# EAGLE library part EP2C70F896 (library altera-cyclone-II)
EP2C70F896 Auto generated by make-symbol-device-package-bsdl.ulp Rev. 19 Tip: Use split-device-symbol.ulp to generate a Device with multiple small symbols! Read HELP. Source: EP2C70F896.BSD
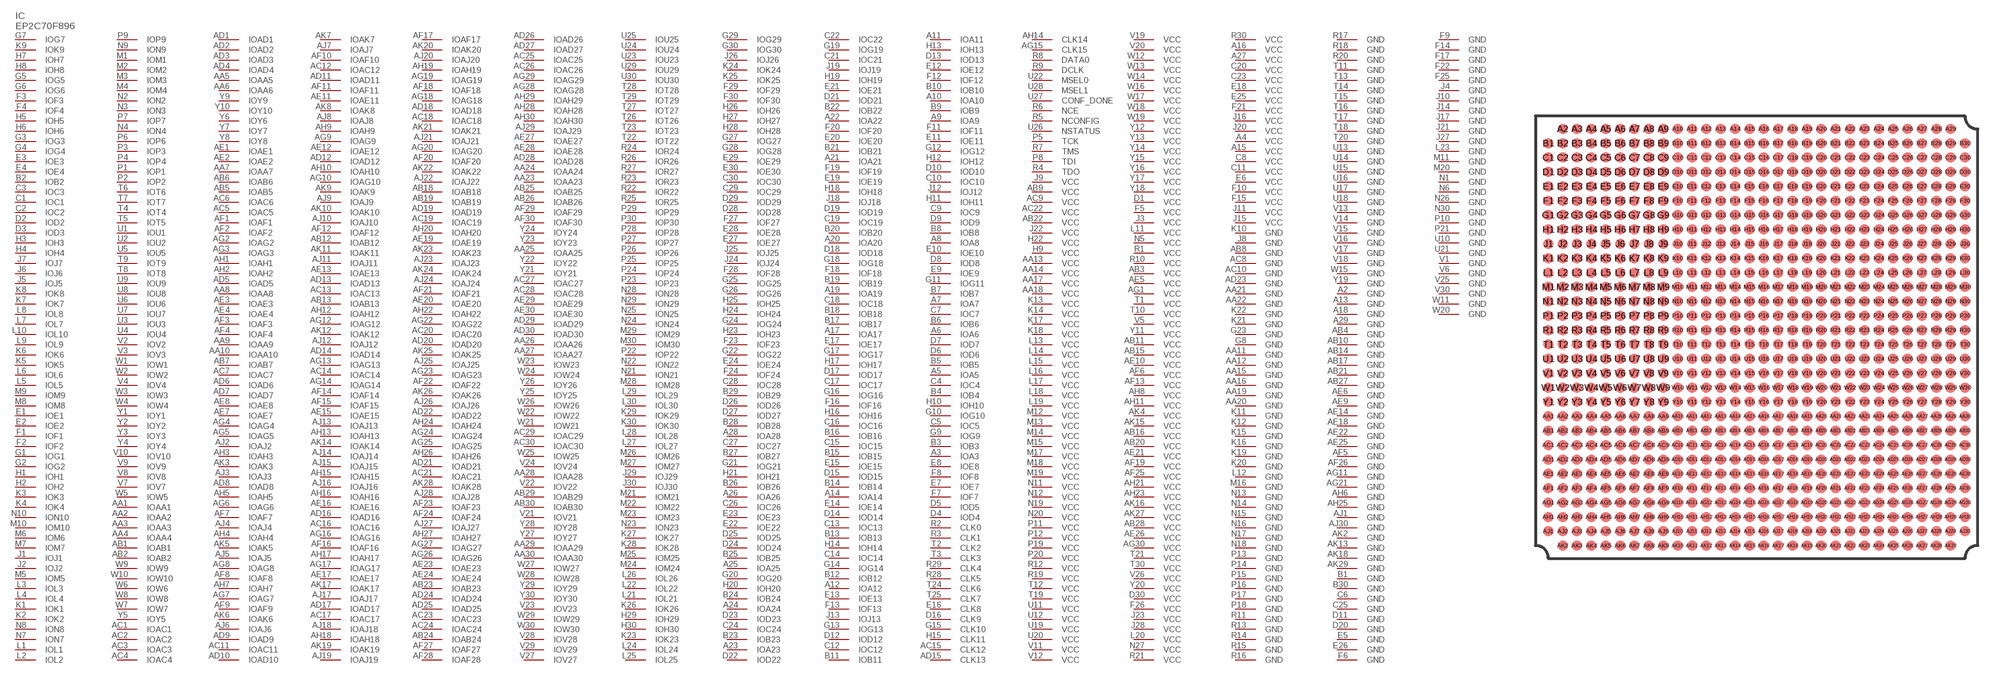
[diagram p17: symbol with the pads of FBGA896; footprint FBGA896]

Designator prefix IC

## EP2C70F896 (MPN: EP2C70F896C8N; OC_FARNELL: 1635092; OC_NEWARK: 51R0573)  [FBGA896]
A2  GND  pwr
A3  IOA3
A4  VCC  pwr
A5  IOA5
A6  IOA6
A7  IOA7
A8  IOA8
A9  IOA9
A10  IOA10
A11  IOA11
A12  IOA12
A13  GND  pwr
A14  IOA14
A15  VCC  pwr
A16  VCC  pwr
A17  IOA17
A18  GND  pwr
A19  IOA19
A20  IOA20
A21  IOA21
A22  IOA22
A23  IOA23
A24  IOA24
A25  IOA25
A26  IOA26
A27  VCC  pwr
A28  IOA28
A29  GND  pwr
AA1  IOAA1
AA2  IOAA2
AA3  IOAA3
AA4  IOAA4
AA5  IOAA5
AA6  IOAA6
AA7  IOAA7
AA8  IOAA8
AA9  IOAA9
AA10  IOAA10
AA11  GND  pwr
AA12  GND  pwr
AA13  VCC  pwr
AA14  VCC  pwr
AA15  GND  pwr
AA16  GND  pwr
AA17  VCC  pwr
AA18  VCC  pwr
AA19  GND  pwr
AA20  GND  pwr
AA21  GND  pwr
AA22  GND  pwr
AA23  IOAA23
AA24  IOAA24
AA25  IOAA25
AA26  IOAA26
AA27  IOAA27
AA28  IOAA28
AA29  IOAA29
AA30  IOAA30
AB1  IOAB1
AB2  IOAB2
AB3  VCC  pwr
AB4  GND  pwr
AB5  IOAB5
AB6  IOAB6
AB7  IOAB7
AB8  GND  pwr
AB9  VCC  pwr
AB10  GND  pwr
AB11  VCC  pwr
AB12  IOAB12
AB13  IOAB13
AB14  GND  pwr
AB15  VCC  pwr
AB16  VCC  pwr
AB17  GND  pwr
AB18  IOAB18
AB19  IOAB19
AB20  VCC  pwr
AB21  GND  pwr
AB22  VCC  pwr
AB23  IOAB23
AB24  IOAB24
AB25  IOAB25
AB26  IOAB26
AB27  GND  pwr
AB28  VCC  pwr
AB29  IOAB29
AB30  IOAB30
AC1  IOAC1
AC2  IOAC2
AC3  IOAC3
AC4  IOAC4
AC5  IOAC5
AC6  IOAC6
AC7  IOAC7
AC8  GND  pwr
AC9  VCC  pwr
AC10  GND  pwr
AC11  IOAC11
AC12  IOAC12
AC13  IOAC13
AC14  IOAC14
AC15  CLK12
AC16  IOAC16
AC17  IOAC17
AC18  IOAC18
AC19  IOAC19
AC20  IOAC20
AC21  IOAC21
AC22  VCC  pwr
AC23  IOAC23
AC24  IOAC24
AC25  IOAC25
AC26  IOAC26
AC27  IOAC27
AC28  IOAC28
AC29  IOAC29
AC30  IOAC30
AD1  IOAD1
AD2  IOAD2
AD3  IOAD3
AD4  IOAD4
AD5  IOAD5
AD6  IOAD6
AD7  IOAD7
AD8  IOAD8
AD9  IOAD9
AD10  IOAD10
AD11  IOAD11
AD12  IOAD12
AD13  IOAD13
AD14  IOAD14
AD15  CLK13
AD16  IOAD16
AD17  IOAD17
AD18  IOAD18
AD19  IOAD19
AD20  IOAD20
AD21  IOAD21
AD22  IOAD22
AD23  GND  pwr
AD24  IOAD24
AD25  IOAD25
AD26  IOAD26
AD27  IOAD27
AD28  IOAD28
AD29  IOAD29
AD30  IOAD30
AE1  IOAE1
AE2  IOAE2
AE3  IOAE3
AE4  IOAE4
AE5  VCC  pwr
AE6  GND  pwr
AE7  IOAE7
AE8  IOAE8
AE9  GND  pwr
AE10  VCC  pwr
AE11  IOAE11
AE12  IOAE12
AE13  IOAE13
AE14  GND  pwr
AE15  IOAE15
AE16  IOAE16
AE17  IOAE17
AE18  GND  pwr
AE19  IOAE19
AE20  IOAE20
AE21  VCC  pwr
AE22  GND  pwr
AE23  IOAE23
AE24  IOAE24
AE25  GND  pwr
AE26  VCC  pwr
AE27  IOAE27
AE28  IOAE28
AE29  IOAE29
AE30  IOAE30
AF1  IOAF1
AF2  IOAF2
AF3  IOAF3
AF4  IOAF4
AF5  GND  pwr
AF6  VCC  pwr
AF7  IOAF7
AF8  IOAF8
AF9  IOAF9
AF10  IOAF10
AF11  IOAF11
AF12  IOAF12
AF13  VCC  pwr
AF14  IOAF14
AF15  IOAF15
AF16  IOAF16
AF17  IOAF17
AF18  IOAF18
AF19  VCC  pwr
AF20  IOAF20
AF21  IOAF21
AF22  IOAF22
AF23  IOAF23
AF24  IOAF24
AF25  VCC  pwr
AF26  GND  pwr
AF27  IOAF27
AF28  IOAF28
AF29  IOAF29
AF30  IOAF30
AG1  VCC  pwr
AG2  IOAG2
AG3  IOAG3
AG4  IOAG4
AG5  IOAG5
AG6  IOAG6
AG7  IOAG7
AG8  IOAG8
AG9  IOAG9
AG10  IOAG10
AG11  GND  pwr
AG12  IOAG12
AG13  IOAG13
AG14  IOAG14
AG15  CLK15
AG16  IOAG16
AG17  IOAG17
AG18  IOAG18
AG19  IOAG19
AG20  IOAG20
AG21  GND  pwr
AG22  IOAG22
AG23  IOAG23
AG24  IOAG24
AG25  IOAG25
AG26  IOAG26
AG27  IOAG27
AG28  IOAG28
AG29  IOAG29
AG30  VCC  pwr
AH1  IOAH1
AH2  IOAH2
AH3  IOAH3
AH4  IOAH4
AH5  IOAH5
AH6  GND  pwr
AH7  IOAH7
AH8  VCC  pwr
AH9  IOAH9
AH10  IOAH10
AH11  VCC  pwr
AH12  IOAH12
AH13  IOAH13
AH14  CLK14
AH15  IOAH15
AH16  IOAH16
AH17  IOAH17
AH18  IOAH18
AH19  IOAH19
AH20  IOAH20
AH21  VCC  pwr
AH22  IOAH22
AH23  VCC  pwr
AH24  IOAH24
AH25  GND  pwr
AH26  IOAH26
AH27  IOAH27
AH28  IOAH28
AH29  IOAH29
AH30  IOAH30
AJ1  GND  pwr
AJ2  IOAJ2
AJ3  IOAJ3
AJ4  IOAJ4
AJ5  IOAJ5
AJ6  IOAJ6
AJ7  IOAJ7
AJ8  IOAJ8
AJ9  IOAJ9
AJ10  IOAJ10
AJ11  IOAJ11
AJ12  IOAJ12
AJ13  IOAJ13
AJ14  IOAJ14
AJ15  IOAJ15
AJ16  IOAJ16
AJ17  IOAJ17
AJ18  IOAJ18
AJ19  IOAJ19
AJ20  IOAJ20
AJ21  IOAJ21
AJ22  IOAJ22
AJ23  IOAJ23
AJ24  IOAJ24
AJ25  IOAJ25
AJ26  IOAJ26
AJ27  IOAJ27
AJ28  IOAJ28
AJ29  IOAJ29
AJ30  GND  pwr
AK2  GND  pwr
AK3  IOAK3
AK4  VCC  pwr
AK5  IOAK5
AK6  IOAK6
AK7  IOAK7
AK8  IOAK8
AK9  IOAK9
AK10  IOAK10
AK11  IOAK11
AK12  IOAK12
AK13  GND  pwr
AK14  IOAK14
AK15  VCC  pwr
AK16  VCC  pwr
AK17  IOAK17
AK18  GND  pwr
AK19  IOAK19
AK20  IOAK20
AK21  IOAK21
AK22  IOAK22
AK23  IOAK23
AK24  IOAK24
AK25  IOAK25
AK26  IOAK26
AK27  VCC  pwr
AK28  IOAK28
AK29  GND  pwr
B1  GND  pwr
B2  IOB2
B3  IOB3
B4  IOB4
B5  IOB5
B6  IOB6
B7  IOB7
B8  IOB8
B9  IOB9
B10  IOB10
B11  IOB11
B12  IOB12
B13  IOB13
B14  IOB14
B15  IOB15
B16  IOB16
B17  IOB17
B18  IOB18
B19  IOB19
B20  IOB20
B21  IOB21
B22  IOB22
B23  IOB23
B24  IOB24
B25  IOB25
B26  IOB26
B27  IOB27
B28  IOB28
B29  IOB29
B30  GND  pwr
C1  IOC1
C2  IOC2
C3  IOC3
C4  IOC4
C5  IOC5
C6  GND  pwr
C7  IOC7
C8  VCC  pwr
C9  IOC9
C10  IOC10
C11  VCC  pwr
C12  IOC12
C13  IOC13
C14  IOC14
C15  IOC15
C16  IOC16
C17  IOC17
C18  IOC18
C19  IOC19
C20  VCC  pwr
C21  IOC21
C22  IOC22
C23  VCC  pwr
C24  IOC24
C25  GND  pwr
C26  IOC26
C27  IOC27
C28  IOC28
C29  IOC29
C30  IOC30
D1  VCC  pwr
D2  IOD2
D3  IOD3
D4  IOD4
D5  IOD5
D6  IOD6
D7  IOD7
D8  IOD8
D9  IOD9
D10  IOD10
D11  GND  pwr
D12  IOD12
D13  IOD13
D14  IOD14
D15  IOD15
D16  CLK9
D17  IOD17
D18  IOD18
D19  IOD19
D20  GND  pwr
D21  IOD21
D22  IOD22
D23  IOD23
D24  IOD24
D25  IOD25
D26  IOD26
D27  IOD27
D28  IOD28
D29  IOD29
D30  VCC  pwr
E1  IOE1
E2  IOE2
E3  IOE3
E4  IOE4
E5  GND  pwr
E6  VCC  pwr
E7  IOE7
E8  IOE8
E9  IOE9
E10  IOE10
E11  IOE11
E12  IOE12
E13  IOE13
E14  IOE14
E15  IOE15
E16  CLK8
E17  IOE17
E18  VCC  pwr
E19  IOE19
E20  IOE20
E21  IOE21
E22  IOE22
E23  IOE23
E24  IOE24
E25  VCC  pwr
E26  GND  pwr
E27  IOE27
E28  IOE28
E29  IOE29
E30  IOE30
F1  IOF1
F2  IOF2
F3  IOF3
F4  IOF4
F5  VCC  pwr
F6  GND  pwr
F7  IOF7
F8  IOF8
F9  GND  pwr
F10  VCC  pwr
F11  IOF11
F12  IOF12
F13  IOF13
F14  GND  pwr
F15  VCC  pwr
F16  IOF16
F17  GND  pwr
F18  IOF18
F19  IOF19
F20  IOF20
F21  VCC  pwr
F22  GND  pwr
F23  IOF23
F24  IOF24
F25  GND  pwr
F26  VCC  pwr
F27  IOF27
F28  IOF28
F29  IOF29
F30  IOF30
G1  IOG1
G2  IOG2
G3  IOG3
G4  IOG4
G5  IOG5
G6  IOG6
G7  IOG7  out
G8  GND  pwr
G9  IOG9
G10  IOG10
G11  IOG11
G12  IOG12
G13  IOG13
G14  IOG14
G15  CLK10
G16  IOG16
G17  IOG17
G18  IOG18
G19  IOG19
G20  IOG20
G21  IOG21
G22  IOG22
G23  GND  pwr
G24  IOG24
G25  IOG25
G26  IOG26
G27  IOG27
G28  IOG28
G29  IOG29
G30  IOG30
H1  IOH1
H2  IOH2
H3  IOH3
H4  IOH4
H5  IOH5
H6  IOH6
H7  IOH7
H8  IOH8
H9  VCC  pwr
H10  IOH10
H11  IOH11
H12  IOH12
H13  IOH13
H14  IOH14
H15  CLK11
H16  IOH16
H17  IOH17
H18  IOH18
H19  IOH19
H20  IOH20
H21  IOH21
H22  VCC  pwr
H23  IOH23
H24  IOH24
H25  IOH25
H26  IOH26
H27  IOH27
H28  IOH28
H29  IOH29
H30  IOH30
J1  IOJ1
J2  IOJ2
J3  VCC  pwr
J4  GND  pwr
J5  IOJ5
J6  IOJ6
J7  IOJ7
J8  GND  pwr
J9  VCC  pwr
J10  GND  pwr
J11  VCC  pwr
J12  IOJ12
J13  IOJ13
J14  GND  pwr
J15  VCC  pwr
J16  VCC  pwr
J17  GND  pwr
J18  IOJ18
J19  IOJ19
J20  VCC  pwr
J21  GND  pwr
J22  VCC  pwr
J23  VCC  pwr
J24  IOJ24
J25  IOJ25
J26  IOJ26
J27  GND  pwr
J28  VCC  pwr
J29  IOJ29
J30  IOJ30
K1  IOK1
K2  IOK2
K3  IOK3
K4  IOK4
K5  IOK5
K6  IOK6
K7  IOK7
K8  IOK8
K9  IOK9  out
K10  GND  pwr
K11  GND  pwr
K12  GND  pwr
K13  VCC  pwr
K14  VCC  pwr
K15  GND  pwr
K16  GND  pwr
K17  VCC  pwr
K18  VCC  pwr
K19  GND  pwr
K20  GND  pwr
K21  GND  pwr
K22  GND  pwr
K23  IOK23
K24  IOK24
K25  IOK25
K26  IOK26
K27  IOK27
K28  IOK28
K29  IOK29
K30  IOK30
L1  IOL1
L2  IOL2
L3  IOL3
L4  IOL4
L5  IOL5
L6  IOL6
L7  IOL7
L8  IOL8
L9  IOL9
L10  IOL10
L11  VCC  pwr
L12  GND  pwr
L13  VCC  pwr
L14  VCC  pwr
L15  VCC  pwr
L16  VCC  pwr
L17  VCC  pwr
L18  VCC  pwr
L19  VCC  pwr
L20  VCC  pwr
L21  IOL21
L22  IOL22
L23  GND  pwr
L24  IOL24
L25  IOL25
L26  IOL26
L27  IOL27
L28  IOL28
L29  IOL29
L30  IOL30
M1  IOM1
M2  IOM2
M3  IOM3
M4  IOM4
M5  IOM5
M6  IOM6
M7  IOM7
M8  IOM8
M9  IOM9
M10  IOM10
M11  GND  pwr
M12  VCC  pwr
M13  VCC  pwr
M14  VCC  pwr
M15  VCC  pwr
M16  GND  pwr
M17  VCC  pwr
M18  VCC  pwr
M19  VCC  pwr
M20  GND  pwr
M21  IOM21
M22  IOM22
M23  IOM23
M24  IOM24
M25  IOM25
M26  IOM26
M27  IOM27
M28  IOM28
M29  IOM29
M30  IOM30
N1  GND  pwr
N2  ION2
N3  ION3
N4  ION4
N5  VCC  pwr
N6  GND  pwr
N7  ION7
N8  ION8
N9  ION9
N10  ION10
N11  VCC  pwr
N12  VCC  pwr
N13  GND  pwr
N14  GND  pwr
N15  GND  pwr
N16  GND  pwr
N17  GND  pwr
N18  GND  pwr
N19  VCC  pwr
N20  VCC  pwr
N21  ION21
N22  ION22
N23  ION23
N24  ION24
N25  ION25
N26  GND  pwr
N27  VCC  pwr
N28  ION28
N29  ION29
N30  GND  pwr
P1  IOP1
P2  IOP2
P3  IOP3
P4  IOP4
P5  TCK  in
P6  IOP6
P7  IOP7
P8  TDI  in
P9  IOP9
P10  GND  pwr
P11  VCC  pwr
P12  VCC  pwr
P13  GND  pwr
P14  GND  pwr
P15  GND  pwr
P16  GND  pwr
P17  GND  pwr
P18  GND  pwr
P19  VCC  pwr
P20  VCC  pwr
P21  GND  pwr
P22  IOP22
P23  IOP23
P24  IOP24
P25  IOP25
P26  IOP26
P27  IOP27
P28  IOP28
P29  IOP29
P30  IOP30
R1  VCC  pwr
R2  CLK0
R3  CLK1
R4  TDO  out
R5  NCONFIG  in
R6  NCE  in
R7  TMS  in
R8  DATA0
R9  DCLK
R10  VCC  pwr
R11  GND  pwr
R12  VCC  pwr
R13  GND  pwr
R14  GND  pwr
R15  GND  pwr
R16  GND  pwr
R17  GND  pwr
R18  GND  pwr
R19  VCC  pwr
R20  GND  pwr
R21  VCC  pwr
R22  IOR22
R23  IOR23
R24  IOR24
R25  IOR25
R26  IOR26
R27  IOR27
R28  CLK5
R29  CLK4
R30  VCC  pwr
T1  VCC  pwr
T2  CLK2
T3  CLK3
T4  IOT4
T5  IOT5
T6  IOT6
T7  IOT7
T8  IOT8
T9  IOT9
T10  VCC  pwr
T11  GND  pwr
T12  VCC  pwr
T13  GND  pwr
T14  GND  pwr
T15  GND  pwr
T16  GND  pwr
T17  GND  pwr
T18  GND  pwr
T19  VCC  pwr
T20  GND  pwr
T21  VCC  pwr
T22  IOT22
T23  IOT23
T24  CLK6
T25  CLK7
T26  IOT26
T27  IOT27
T28  IOT28
T29  IOT29
T30  VCC  pwr
U1  IOU1
U2  IOU2
U3  IOU3
U4  IOU4
U5  IOU5
U6  IOU6
U7  IOU7
U8  IOU8
U9  IOU9
U10  GND  pwr
U11  VCC  pwr
U12  VCC  pwr
U13  GND  pwr
U14  GND  pwr
U15  GND  pwr
U16  GND  pwr
U17  GND  pwr
U18  GND  pwr
U19  VCC  pwr
U20  VCC  pwr
U21  GND  pwr
U22  MSEL0  in
U23  IOU23
U24  IOU24
U25  IOU25
U26  NSTATUS  in
U27  CONF_DONE  in
U28  MSEL1  in
U29  IOU29
U30  IOU30
V1  GND  pwr
V2  IOV2
V3  IOV3
V4  IOV4
V5  VCC  pwr
V6  GND  pwr
V7  IOV7
V8  IOV8
V9  IOV9
V10  IOV10
V11  VCC  pwr
V12  VCC  pwr
V13  GND  pwr
V14  GND  pwr
V15  GND  pwr
V16  GND  pwr
V17  GND  pwr
V18  GND  pwr
V19  VCC  pwr
V20  VCC  pwr
V21  IOV21
V22  IOV22
V23  IOV23
V24  IOV24
V25  GND  pwr
V26  VCC  pwr
V27  IOV27
V28  IOV28
V29  IOV29
V30  GND  pwr
W1  IOW1
W2  IOW2
W3  IOW3
W4  IOW4
W5  IOW5
W6  IOW6
W7  IOW7
W8  IOW8
W9  IOW9
W10  IOW10
W11  GND  pwr
W12  VCC  pwr
W13  VCC  pwr
W14  VCC  pwr
W15  GND  pwr
W16  VCC  pwr
W17  VCC  pwr
W18  VCC  pwr
W19  VCC  pwr
W20  GND  pwr
W21  IOW21
W22  IOW22
W23  IOW23
W24  IOW24
W25  IOW25
W26  IOW26
W27  IOW27
W28  IOW28
W29  IOW29
W30  IOW30
Y1  IOY1
Y2  IOY2
Y3  IOY3
Y4  IOY4
Y5  IOY5
Y6  IOY6
Y7  IOY7
Y8  IOY8
Y9  IOY9
Y10  IOY10
Y11  VCC  pwr
Y12  VCC  pwr
Y13  VCC  pwr
Y14  VCC  pwr
Y15  VCC  pwr
Y16  VCC  pwr
Y17  VCC  pwr
Y18  VCC  pwr
Y19  GND  pwr
Y20  VCC  pwr
Y21  IOY21
Y22  IOY22
Y23  IOY23
Y24  IOY24
Y25  IOY25
Y26  IOY26
Y27  IOY27
Y28  IOY28
Y29  IOY29
Y30  IOY30

## Footprint FBGA896 (pad centres in mm)
EP2C70F896 Auto generated by make-symbol-device-package-bsdl.ulp Rev. 19 Source: EP2C70F896.BSD www.altera.com .. cyc2_cii51015.pdf
smd 0.7 x 0.7: A2 -13.5,14.5; A3 -12.5,14.5; A4 -11.5,14.5; A5 -10.5,14.5; A6 -9.5,14.5; A7 -8.5,14.5; A8 -7.5,14.5; A9 -6.5,14.5; A10 -5.5,14.5; A11 -4.5,14.5; A12 -3.5,14.5; A13 -2.5,14.5; A14 -1.5,14.5; A15 -0.5,14.5; A16 0.5,14.5; A17 1.5,14.5; A18 2.5,14.5; A19 3.5,14.5; A20 4.5,14.5; A21 5.5,14.5; A22 6.5,14.5; A23 7.5,14.5; A24 8.5,14.5; A25 9.5,14.5; A26 10.5,14.5; A27 11.5,14.5; A28 12.5,14.5; A29 13.5,14.5; AA1 -14.5,-5.5; AA2 -13.5,-5.5; AA3 -12.5,-5.5; AA4 -11.5,-5.5; AA5 -10.5,-5.5; AA6 -9.5,-5.5; AA7 -8.5,-5.5; AA8 -7.5,-5.5; AA9 -6.5,-5.5; AA10 -5.5,-5.5; AA11 -4.5,-5.5; AA12 -3.5,-5.5; AA13 -2.5,-5.5; AA14 -1.5,-5.5; AA15 -0.5,-5.5; AA16 0.5,-5.5; AA17 1.5,-5.5; AA18 2.5,-5.5; AA19 3.5,-5.5; AA20 4.5,-5.5; AA21 5.5,-5.5; AA22 6.5,-5.5; AA23 7.5,-5.5; AA24 8.5,-5.5; AA25 9.5,-5.5; AA26 10.5,-5.5; AA27 11.5,-5.5; AA28 12.5,-5.5; AA29 13.5,-5.5; AA30 14.5,-5.5; AB1 -14.5,-6.5; AB2 -13.5,-6.5; AB3 -12.5,-6.5; AB4 -11.5,-6.5; AB5 -10.5,-6.5; AB6 -9.5,-6.5; AB7 -8.5,-6.5; AB8 -7.5,-6.5; AB9 -6.5,-6.5; AB10 -5.5,-6.5; AB11 -4.5,-6.5; AB12 -3.5,-6.5; AB13 -2.5,-6.5; AB14 -1.5,-6.5; AB15 -0.5,-6.5; AB16 0.5,-6.5; AB17 1.5,-6.5; AB18 2.5,-6.5; AB19 3.5,-6.5; AB20 4.5,-6.5; AB21 5.5,-6.5; AB22 6.5,-6.5; AB23 7.5,-6.5; AB24 8.5,-6.5; AB25 9.5,-6.5; AB26 10.5,-6.5; AB27 11.5,-6.5; AB28 12.5,-6.5; AB29 13.5,-6.5; AB30 14.5,-6.5; AC1 -14.5,-7.5; AC2 -13.5,-7.5; AC3 -12.5,-7.5; AC4 -11.5,-7.5; AC5 -10.5,-7.5; AC6 -9.5,-7.5; AC7 -8.5,-7.5; AC8 -7.5,-7.5; AC9 -6.5,-7.5; AC10 -5.5,-7.5; AC11 -4.5,-7.5; AC12 -3.5,-7.5; AC13 -2.5,-7.5; AC14 -1.5,-7.5; AC15 -0.5,-7.5; AC16 0.5,-7.5; AC17 1.5,-7.5; AC18 2.5,-7.5; AC19 3.5,-7.5; AC20 4.5,-7.5; AC21 5.5,-7.5; AC22 6.5,-7.5; AC23 7.5,-7.5; AC24 8.5,-7.5; AC25 9.5,-7.5; AC26 10.5,-7.5; AC27 11.5,-7.5; AC28 12.5,-7.5; AC29 13.5,-7.5; AC30 14.5,-7.5; AD1 -14.5,-8.5; AD2 -13.5,-8.5; AD3 -12.5,-8.5; AD4 -11.5,-8.5; AD5 -10.5,-8.5; AD6 -9.5,-8.5; AD7 -8.5,-8.5; AD8 -7.5,-8.5; AD9 -6.5,-8.5; AD10 -5.5,-8.5; AD11 -4.5,-8.5; AD12 -3.5,-8.5; AD13 -2.5,-8.5; AD14 -1.5,-8.5; AD15 -0.5,-8.5; AD16 0.5,-8.5; AD17 1.5,-8.5; AD18 2.5,-8.5; AD19 3.5,-8.5; AD20 4.5,-8.5; AD21 5.5,-8.5; AD22 6.5,-8.5; AD23 7.5,-8.5; AD24 8.5,-8.5; AD25 9.5,-8.5; AD26 10.5,-8.5; AD27 11.5,-8.5; AD28 12.5,-8.5; AD29 13.5,-8.5; AD30 14.5,-8.5; AE1 -14.5,-9.5; AE2 -13.5,-9.5; AE3 -12.5,-9.5; AE4 -11.5,-9.5; AE5 -10.5,-9.5; AE6 -9.5,-9.5; AE7 -8.5,-9.5; AE8 -7.5,-9.5; AE9 -6.5,-9.5; AE10 -5.5,-9.5; AE11 -4.5,-9.5; AE12 -3.5,-9.5; AE13 -2.5,-9.5; AE14 -1.5,-9.5; AE15 -0.5,-9.5; AE16 0.5,-9.5; AE17 1.5,-9.5; AE18 2.5,-9.5; AE19 3.5,-9.5; AE20 4.5,-9.5; AE21 5.5,-9.5; AE22 6.5,-9.5; AE23 7.5,-9.5; AE24 8.5,-9.5; AE25 9.5,-9.5; AE26 10.5,-9.5; AE27 11.5,-9.5; AE28 12.5,-9.5; AE29 13.5,-9.5; AE30 14.5,-9.5; AF1 -14.5,-10.5; AF2 -13.5,-10.5; AF3 -12.5,-10.5; AF4 -11.5,-10.5; AF5 -10.5,-10.5; AF6 -9.5,-10.5; AF7 -8.5,-10.5; AF8 -7.5,-10.5; AF9 -6.5,-10.5; AF10 -5.5,-10.5; AF11 -4.5,-10.5; AF12 -3.5,-10.5; AF13 -2.5,-10.5; AF14 -1.5,-10.5; AF15 -0.5,-10.5; AF16 0.5,-10.5; AF17 1.5,-10.5; AF18 2.5,-10.5; AF19 3.5,-10.5; AF20 4.5,-10.5; AF21 5.5,-10.5; AF22 6.5,-10.5; AF23 7.5,-10.5; AF24 8.5,-10.5; AF25 9.5,-10.5; AF26 10.5,-10.5; AF27 11.5,-10.5; AF28 12.5,-10.5; AF29 13.5,-10.5; AF30 14.5,-10.5; AG1 -14.5,-11.5; AG2 -13.5,-11.5; AG3 -12.5,-11.5; AG4 -11.5,-11.5; AG5 -10.5,-11.5; AG6 -9.5,-11.5; AG7 -8.5,-11.5; AG8 -7.5,-11.5; AG9 -6.5,-11.5; AG10 -5.5,-11.5; AG11 -4.5,-11.5; AG12 -3.5,-11.5; AG13 -2.5,-11.5; AG14 -1.5,-11.5; AG15 -0.5,-11.5; AG16 0.5,-11.5; AG17 1.5,-11.5; AG18 2.5,-11.5; AG19 3.5,-11.5; AG20 4.5,-11.5; AG21 5.5,-11.5; AG22 6.5,-11.5; AG23 7.5,-11.5; AG24 8.5,-11.5; AG25 9.5,-11.5; AG26 10.5,-11.5; AG27 11.5,-11.5; AG28 12.5,-11.5; AG29 13.5,-11.5; AG30 14.5,-11.5; AH1 -14.5,-12.5; AH2 -13.5,-12.5; AH3 -12.5,-12.5; AH4 -11.5,-12.5; AH5 -10.5,-12.5; AH6 -9.5,-12.5; AH7 -8.5,-12.5; AH8 -7.5,-12.5; AH9 -6.5,-12.5; AH10 -5.5,-12.5; AH11 -4.5,-12.5; AH12 -3.5,-12.5; AH13 -2.5,-12.5; AH14 -1.5,-12.5; AH15 -0.5,-12.5; AH16 0.5,-12.5; AH17 1.5,-12.5; AH18 2.5,-12.5; AH19 3.5,-12.5; AH20 4.5,-12.5; AH21 5.5,-12.5; AH22 6.5,-12.5; AH23 7.5,-12.5; AH24 8.5,-12.5; AH25 9.5,-12.5; AH26 10.5,-12.5; AH27 11.5,-12.5; AH28 12.5,-12.5; AH29 13.5,-12.5; AH30 14.5,-12.5; AJ1 -14.5,-13.5; AJ2 -13.5,-13.5; AJ3 -12.5,-13.5; AJ4 -11.5,-13.5; AJ5 -10.5,-13.5; AJ6 -9.5,-13.5; AJ7 -8.5,-13.5; AJ8 -7.5,-13.5; AJ9 -6.5,-13.5; AJ10 -5.5,-13.5; AJ11 -4.5,-13.5; AJ12 -3.5,-13.5; AJ13 -2.5,-13.5; AJ14 -1.5,-13.5; AJ15 -0.5,-13.5; AJ16 0.5,-13.5; AJ17 1.5,-13.5; AJ18 2.5,-13.5; AJ19 3.5,-13.5; AJ20 4.5,-13.5; AJ21 5.5,-13.5; AJ22 6.5,-13.5; AJ23 7.5,-13.5; AJ24 8.5,-13.5; AJ25 9.5,-13.5; AJ26 10.5,-13.5; AJ27 11.5,-13.5; AJ28 12.5,-13.5; AJ29 13.5,-13.5; AJ30 14.5,-13.5; AK2 -13.5,-14.5; AK3 -12.5,-14.5; AK4 -11.5,-14.5; AK5 -10.5,-14.5; AK6 -9.5,-14.5; AK7 -8.5,-14.5; AK8 -7.5,-14.5; AK9 -6.5,-14.5; AK10 -5.5,-14.5; AK11 -4.5,-14.5; AK12 -3.5,-14.5; AK13 -2.5,-14.5; AK14 -1.5,-14.5; AK15 -0.5,-14.5; AK16 0.5,-14.5; AK17 1.5,-14.5; AK18 2.5,-14.5; AK19 3.5,-14.5; AK20 4.5,-14.5; AK21 5.5,-14.5; AK22 6.5,-14.5; AK23 7.5,-14.5; AK24 8.5,-14.5; AK25 9.5,-14.5; AK26 10.5,-14.5; AK27 11.5,-14.5; AK28 12.5,-14.5; AK29 13.5,-14.5; B1 -14.5,13.5; B2 -13.5,13.5; B3 -12.5,13.5; B4 -11.5,13.5; B5 -10.5,13.5; B6 -9.5,13.5; B7 -8.5,13.5; B8 -7.5,13.5; B9 -6.5,13.5; B10 -5.5,13.5; B11 -4.5,13.5; B12 -3.5,13.5; B13 -2.5,13.5; B14 -1.5,13.5; B15 -0.5,13.5; B16 0.5,13.5; B17 1.5,13.5; B18 2.5,13.5; B19 3.5,13.5; B20 4.5,13.5; B21 5.5,13.5; B22 6.5,13.5; B23 7.5,13.5; B24 8.5,13.5; B25 9.5,13.5; B26 10.5,13.5; B27 11.5,13.5; B28 12.5,13.5; B29 13.5,13.5; B30 14.5,13.5; C1 -14.5,12.5; C2 -13.5,12.5; C3 -12.5,12.5; C4 -11.5,12.5; C5 -10.5,12.5; C6 -9.5,12.5; C7 -8.5,12.5; C8 -7.5,12.5; C9 -6.5,12.5; C10 -5.5,12.5; C11 -4.5,12.5; C12 -3.5,12.5; C13 -2.5,12.5; C14 -1.5,12.5; C15 -0.5,12.5; C16 0.5,12.5; C17 1.5,12.5; C18 2.5,12.5; C19 3.5,12.5; C20 4.5,12.5; C21 5.5,12.5; C22 6.5,12.5; C23 7.5,12.5; C24 8.5,12.5; C25 9.5,12.5; C26 10.5,12.5; C27 11.5,12.5; C28 12.5,12.5; C29 13.5,12.5; C30 14.5,12.5; D1 -14.5,11.5; D2 -13.5,11.5; D3 -12.5,11.5; D4 -11.5,11.5; D5 -10.5,11.5; D6 -9.5,11.5; D7 -8.5,11.5; D8 -7.5,11.5; D9 -6.5,11.5; D10 -5.5,11.5; D11 -4.5,11.5; D12 -3.5,11.5; D13 -2.5,11.5; D14 -1.5,11.5; D15 -0.5,11.5; D16 0.5,11.5; D17 1.5,11.5; D18 2.5,11.5; D19 3.5,11.5; D20 4.5,11.5; D21 5.5,11.5; D22 6.5,11.5; D23 7.5,11.5; D24 8.5,11.5; D25 9.5,11.5; D26 10.5,11.5; D27 11.5,11.5; D28 12.5,11.5; D29 13.5,11.5; D30 14.5,11.5; E1 -14.5,10.5; E2 -13.5,10.5; E3 -12.5,10.5; E4 -11.5,10.5; E5 -10.5,10.5; E6 -9.5,10.5; E7 -8.5,10.5; E8 -7.5,10.5; E9 -6.5,10.5; E10 -5.5,10.5; E11 -4.5,10.5; E12 -3.5,10.5; E13 -2.5,10.5; E14 -1.5,10.5; E15 -0.5,10.5; E16 0.5,10.5; E17 1.5,10.5; E18 2.5,10.5; E19 3.5,10.5; E20 4.5,10.5; E21 5.5,10.5; E22 6.5,10.5; E23 7.5,10.5; E24 8.5,10.5; E25 9.5,10.5; E26 10.5,10.5; E27 11.5,10.5; E28 12.5,10.5; E29 13.5,10.5; E30 14.5,10.5; F1 -14.5,9.5; F2 -13.5,9.5; F3 -12.5,9.5; F4 -11.5,9.5; F5 -10.5,9.5; F6 -9.5,9.5; F7 -8.5,9.5; F8 -7.5,9.5; F9 -6.5,9.5; F10 -5.5,9.5; F11 -4.5,9.5; F12 -3.5,9.5; F13 -2.5,9.5; F14 -1.5,9.5; F15 -0.5,9.5; F16 0.5,9.5; F17 1.5,9.5; F18 2.5,9.5; F19 3.5,9.5; F20 4.5,9.5; F21 5.5,9.5; F22 6.5,9.5; F23 7.5,9.5; F24 8.5,9.5; F25 9.5,9.5; F26 10.5,9.5; F27 11.5,9.5; F28 12.5,9.5; F29 13.5,9.5; F30 14.5,9.5; G1 -14.5,8.5; G2 -13.5,8.5; G3 -12.5,8.5; G4 -11.5,8.5; G5 -10.5,8.5; G6 -9.5,8.5; G7 -8.5,8.5; G8 -7.5,8.5; G9 -6.5,8.5; G10 -5.5,8.5; G11 -4.5,8.5; G12 -3.5,8.5; G13 -2.5,8.5; G14 -1.5,8.5; G15 -0.5,8.5; G16 0.5,8.5; G17 1.5,8.5; G18 2.5,8.5; G19 3.5,8.5; G20 4.5,8.5; G21 5.5,8.5; G22 6.5,8.5; G23 7.5,8.5; G24 8.5,8.5; G25 9.5,8.5; G26 10.5,8.5; G27 11.5,8.5; G28 12.5,8.5; G29 13.5,8.5; G30 14.5,8.5; H1 -14.5,7.5; H2 -13.5,7.5; H3 -12.5,7.5; H4 -11.5,7.5; H5 -10.5,7.5; H6 -9.5,7.5; H7 -8.5,7.5; H8 -7.5,7.5; H9 -6.5,7.5; H10 -5.5,7.5; H11 -4.5,7.5; H12 -3.5,7.5; H13 -2.5,7.5; H14 -1.5,7.5; H15 -0.5,7.5; H16 0.5,7.5; H17 1.5,7.5; H18 2.5,7.5; H19 3.5,7.5; H20 4.5,7.5; H21 5.5,7.5; H22 6.5,7.5; H23 7.5,7.5; H24 8.5,7.5; H25 9.5,7.5; H26 10.5,7.5; H27 11.5,7.5; H28 12.5,7.5; H29 13.5,7.5; H30 14.5,7.5; J1 -14.5,6.5; J2 -13.5,6.5; J3 -12.5,6.5; J4 -11.5,6.5; J5 -10.5,6.5; J6 -9.5,6.5; J7 -8.5,6.5; J8 -7.5,6.5; J9 -6.5,6.5; J10 -5.5,6.5; J11 -4.5,6.5; J12 -3.5,6.5; J13 -2.5,6.5; J14 -1.5,6.5; J15 -0.5,6.5; J16 0.5,6.5; J17 1.5,6.5; J18 2.5,6.5; J19 3.5,6.5; J20 4.5,6.5; J21 5.5,6.5; J22 6.5,6.5; J23 7.5,6.5; J24 8.5,6.5; J25 9.5,6.5; J26 10.5,6.5; J27 11.5,6.5; J28 12.5,6.5; J29 13.5,6.5; J30 14.5,6.5; K1 -14.5,5.5; K2 -13.5,5.5; K3 -12.5,5.5; K4 -11.5,5.5; K5 -10.5,5.5; K6 -9.5,5.5; K7 -8.5,5.5; K8 -7.5,5.5; K9 -6.5,5.5; K10 -5.5,5.5; K11 -4.5,5.5; K12 -3.5,5.5; K13 -2.5,5.5; K14 -1.5,5.5; K15 -0.5,5.5; K16 0.5,5.5; K17 1.5,5.5; K18 2.5,5.5; K19 3.5,5.5; K20 4.5,5.5; K21 5.5,5.5; K22 6.5,5.5; K23 7.5,5.5; K24 8.5,5.5; K25 9.5,5.5; K26 10.5,5.5; K27 11.5,5.5; K28 12.5,5.5; K29 13.5,5.5; K30 14.5,5.5; L1 -14.5,4.5; L2 -13.5,4.5; L3 -12.5,4.5; L4 -11.5,4.5; L5 -10.5,4.5; L6 -9.5,4.5; L7 -8.5,4.5; L8 -7.5,4.5; L9 -6.5,4.5; L10 -5.5,4.5; L11 -4.5,4.5; L12 -3.5,4.5; L13 -2.5,4.5; L14 -1.5,4.5; L15 -0.5,4.5; L16 0.5,4.5; L17 1.5,4.5; L18 2.5,4.5; L19 3.5,4.5; L20 4.5,4.5; L21 5.5,4.5; L22 6.5,4.5; L23 7.5,4.5; L24 8.5,4.5; L25 9.5,4.5; L26 10.5,4.5; L27 11.5,4.5; L28 12.5,4.5; L29 13.5,4.5; L30 14.5,4.5; M1 -14.5,3.5; M2 -13.5,3.5; M3 -12.5,3.5; M4 -11.5,3.5; M5 -10.5,3.5; M6 -9.5,3.5; M7 -8.5,3.5; M8 -7.5,3.5; M9 -6.5,3.5; M10 -5.5,3.5; M11 -4.5,3.5; M12 -3.5,3.5; M13 -2.5,3.5; M14 -1.5,3.5; M15 -0.5,3.5; M16 0.5,3.5; M17 1.5,3.5; M18 2.5,3.5; M19 3.5,3.5; M20 4.5,3.5; M21 5.5,3.5; M22 6.5,3.5; M23 7.5,3.5; M24 8.5,3.5; M25 9.5,3.5; M26 10.5,3.5; M27 11.5,3.5; M28 12.5,3.5; M29 13.5,3.5; M30 14.5,3.5; N1 -14.5,2.5; N2 -13.5,2.5; N3 -12.5,2.5; N4 -11.5,2.5; N5 -10.5,2.5; N6 -9.5,2.5; N7 -8.5,2.5; N8 -7.5,2.5; N9 -6.5,2.5; N10 -5.5,2.5; N11 -4.5,2.5; N12 -3.5,2.5; N13 -2.5,2.5; N14 -1.5,2.5; N15 -0.5,2.5; N16 0.5,2.5; N17 1.5,2.5; N18 2.5,2.5; N19 3.5,2.5; N20 4.5,2.5; N21 5.5,2.5; N22 6.5,2.5; N23 7.5,2.5; N24 8.5,2.5; N25 9.5,2.5; N26 10.5,2.5; N27 11.5,2.5; N28 12.5,2.5; N29 13.5,2.5; N30 14.5,2.5; P1 -14.5,1.5; P2 -13.5,1.5; P3 -12.5,1.5; P4 -11.5,1.5; P5 -10.5,1.5; P6 -9.5,1.5; P7 -8.5,1.5; P8 -7.5,1.5; P9 -6.5,1.5; P10 -5.5,1.5; P11 -4.5,1.5; P12 -3.5,1.5; P13 -2.5,1.5; P14 -1.5,1.5; P15 -0.5,1.5; P16 0.5,1.5; P17 1.5,1.5; P18 2.5,1.5; P19 3.5,1.5; P20 4.5,1.5; P21 5.5,1.5; P22 6.5,1.5; P23 7.5,1.5; P24 8.5,1.5; P25 9.5,1.5; P26 10.5,1.5; P27 11.5,1.5; P28 12.5,1.5; P29 13.5,1.5; P30 14.5,1.5; R1 -14.5,0.5; R2 -13.5,0.5; R3 -12.5,0.5; R4 -11.5,0.5; R5 -10.5,0.5; R6 -9.5,0.5; R7 -8.5,0.5; R8 -7.5,0.5; R9 -6.5,0.5; R10 -5.5,0.5; R11 -4.5,0.5; R12 -3.5,0.5; R13 -2.5,0.5; R14 -1.5,0.5; R15 -0.5,0.5; R16 0.5,0.5; R17 1.5,0.5; R18 2.5,0.5; R19 3.5,0.5; R20 4.5,0.5; R21 5.5,0.5; R22 6.5,0.5; R23 7.5,0.5; R24 8.5,0.5; R25 9.5,0.5; R26 10.5,0.5; R27 11.5,0.5; R28 12.5,0.5; R29 13.5,0.5; R30 14.5,0.5; T1 -14.5,-0.5; T2 -13.5,-0.5; T3 -12.5,-0.5; T4 -11.5,-0.5; T5 -10.5,-0.5; T6 -9.5,-0.5; T7 -8.5,-0.5; T8 -7.5,-0.5; T9 -6.5,-0.5; T10 -5.5,-0.5; T11 -4.5,-0.5; T12 -3.5,-0.5; T13 -2.5,-0.5; T14 -1.5,-0.5; T15 -0.5,-0.5; T16 0.5,-0.5; T17 1.5,-0.5; T18 2.5,-0.5; T19 3.5,-0.5; T20 4.5,-0.5; T21 5.5,-0.5; T22 6.5,-0.5; T23 7.5,-0.5; T24 8.5,-0.5; T25 9.5,-0.5; T26 10.5,-0.5; T27 11.5,-0.5; T28 12.5,-0.5; T29 13.5,-0.5; T30 14.5,-0.5; U1 -14.5,-1.5; U2 -13.5,-1.5; U3 -12.5,-1.5; U4 -11.5,-1.5; U5 -10.5,-1.5; U6 -9.5,-1.5; U7 -8.5,-1.5; U8 -7.5,-1.5; U9 -6.5,-1.5; U10 -5.5,-1.5; U11 -4.5,-1.5; U12 -3.5,-1.5; U13 -2.5,-1.5; U14 -1.5,-1.5; U15 -0.5,-1.5; U16 0.5,-1.5; U17 1.5,-1.5; U18 2.5,-1.5; U19 3.5,-1.5; U20 4.5,-1.5; U21 5.5,-1.5; U22 6.5,-1.5; U23 7.5,-1.5; U24 8.5,-1.5; U25 9.5,-1.5; U26 10.5,-1.5; U27 11.5,-1.5; U28 12.5,-1.5; U29 13.5,-1.5; U30 14.5,-1.5; V1 -14.5,-2.5; V2 -13.5,-2.5; V3 -12.5,-2.5; V4 -11.5,-2.5; V5 -10.5,-2.5; V6 -9.5,-2.5; V7 -8.5,-2.5; V8 -7.5,-2.5; V9 -6.5,-2.5; V10 -5.5,-2.5; V11 -4.5,-2.5; V12 -3.5,-2.5; V13 -2.5,-2.5; V14 -1.5,-2.5; V15 -0.5,-2.5; V16 0.5,-2.5; V17 1.5,-2.5; V18 2.5,-2.5; V19 3.5,-2.5; V20 4.5,-2.5; V21 5.5,-2.5; V22 6.5,-2.5; V23 7.5,-2.5; V24 8.5,-2.5; V25 9.5,-2.5; V26 10.5,-2.5; V27 11.5,-2.5; V28 12.5,-2.5; V29 13.5,-2.5; V30 14.5,-2.5; W1 -14.5,-3.5; W2 -13.5,-3.5; W3 -12.5,-3.5; W4 -11.5,-3.5; W5 -10.5,-3.5; W6 -9.5,-3.5; W7 -8.5,-3.5; W8 -7.5,-3.5; W9 -6.5,-3.5; W10 -5.5,-3.5; W11 -4.5,-3.5; W12 -3.5,-3.5; W13 -2.5,-3.5; W14 -1.5,-3.5; W15 -0.5,-3.5; W16 0.5,-3.5; W17 1.5,-3.5; W18 2.5,-3.5; W19 3.5,-3.5; W20 4.5,-3.5; W21 5.5,-3.5; W22 6.5,-3.5; W23 7.5,-3.5; W24 8.5,-3.5; W25 9.5,-3.5; W26 10.5,-3.5; W27 11.5,-3.5; W28 12.5,-3.5; W29 13.5,-3.5; W30 14.5,-3.5; Y1 -14.5,-4.5; Y2 -13.5,-4.5; Y3 -12.5,-4.5; Y4 -11.5,-4.5; Y5 -10.5,-4.5; Y6 -9.5,-4.5; Y7 -8.5,-4.5; Y8 -7.5,-4.5; Y9 -6.5,-4.5; Y10 -5.5,-4.5; Y11 -4.5,-4.5; Y12 -3.5,-4.5; Y13 -2.5,-4.5; Y14 -1.5,-4.5; Y15 -0.5,-4.5; Y16 0.5,-4.5; Y17 1.5,-4.5; Y18 2.5,-4.5; Y19 3.5,-4.5; Y20 4.5,-4.5; Y21 5.5,-4.5; Y22 6.5,-4.5; Y23 7.5,-4.5; Y24 8.5,-4.5; Y25 9.5,-4.5; Y26 10.5,-4.5; Y27 11.5,-4.5; Y28 12.5,-4.5; Y29 13.5,-4.5; Y30 14.5,-4.5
